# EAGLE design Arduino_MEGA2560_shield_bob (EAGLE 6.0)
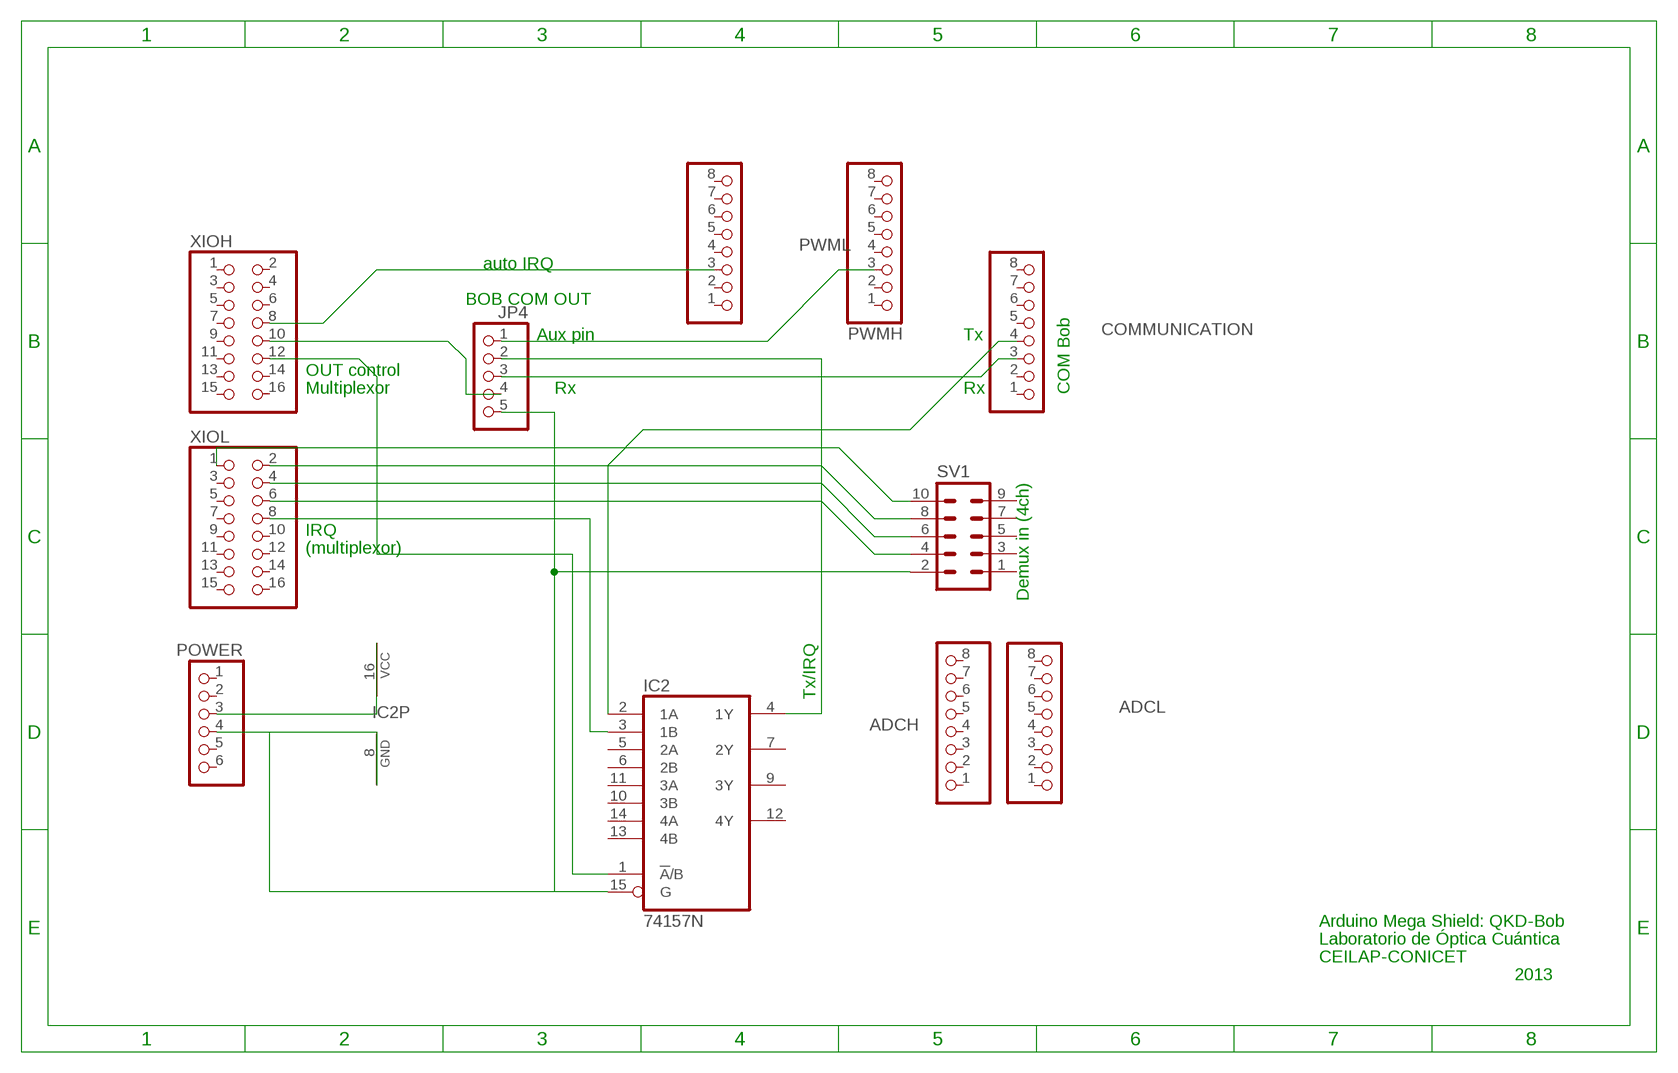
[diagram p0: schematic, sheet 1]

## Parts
ADCH  PINHD-1X8  [1X08]
ADCL  PINHD-1X8  [1X08]
COMMUNICATION  PINHD-1X8  [1X08]
IC2  74157N  [DIL16]
JP4  PINHD-1X5  [1X05]
POWER  PINHD-1X6  [1X06]
PWMH  PINHD-1X8  [1X08]
PWML  PINHD-1X8  [1X08]
SV1  ML10  [ML10]
XIOH  PINHD-2X8  [2X08]
XIOL  PINHD-2X8  [2X08]

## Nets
GND: IC2.8(GND) IC2.15(G) JP4.5 POWER.4 SV1.2
N$1: IC2.3(1B) XIOL.8
N$2: IC2.4(1Y) JP4.2
N$3: IC2.1(!A!/B) XIOH.12
N$4: IC2.16(VCC) POWER.3
N$5: SV1.10 XIOL.1
N$6: JP4.4 XIOH.10
N$7: JP4.1 PWMH.3
N$8: SV1.8 XIOL.2
N$9: COMMUNICATION.4 IC2.2(1A)
N$10: COMMUNICATION.3 JP4.3
N$11: SV1.6 XIOL.4
N$12: SV1.4 XIOL.6
N$13: PWML.3 XIOH.8
Unconnected: ADCH.1 ADCH.2 ADCH.3 ADCH.4 ADCH.5 ADCH.6 ADCH.7 ADCH.8 ADCL.1 ADCL.2 ADCL.3 ADCL.4 ADCL.5 ADCL.6 ADCL.7 ADCL.8 COMMUNICATION.1 COMMUNICATION.2 COMMUNICATION.5 COMMUNICATION.6 COMMUNICATION.7 COMMUNICATION.8 IC2.5(2A) IC2.6(2B) IC2.7(2Y) IC2.9(3Y) IC2.10(3B) IC2.11(3A) IC2.12(4Y) IC2.13(4B) IC2.14(4A) POWER.1 POWER.2 POWER.5 POWER.6 PWMH.1 PWMH.2 PWMH.4 PWMH.5 PWMH.6 PWMH.7 PWMH.8 PWML.1 PWML.2 PWML.4 PWML.5 PWML.6 PWML.7 PWML.8 SV1.1 SV1.3 SV1.5 SV1.7 SV1.9 XIOH.1 XIOH.2 XIOH.3 XIOH.4 XIOH.5 XIOH.6 XIOH.7 XIOH.9 XIOH.11 XIOH.13 XIOH.14 XIOH.15 XIOH.16 XIOL.3 XIOL.5 XIOL.7 XIOL.9 XIOL.10 XIOL.11 XIOL.12 XIOL.13 XIOL.14 XIOL.15 XIOL.16

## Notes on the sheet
- auto IRQ
- BOB COM OUT
- Aux pin | Tx
- OUT control
- Multiplexor | Rx | Rx | COM Bob
- Demux in (4ch)
- IRQ
- (multiplexor)
- Tx/IRQ
- Arduino Mega Shield: QKD-Bob
- Laboratorio de Óptica Cuántica
- CEILAP-CONICET
- 2013

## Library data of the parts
ADCH ADCL COMMUNICATION PWMH PWML = pinhead:PINHD-1X8: PIN HEADER
IC2 = 74xx-us:74*157: Quadruple 2-line to 1-line data SELECTOR/MULTIPLEXER
JP4 = pinhead:PINHD-1X5: PIN HEADER
POWER = pinhead:PINHD-1X6: PIN HEADER
SV1 = con-harting-ml:ML10: HARTING; OC_FARNELL: unknown; OC_NEWARK: unknown
XIOH XIOL = pinhead:PINHD-2X8: PIN HEADER

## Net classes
0 default: width 0.152 mm, drill 0.305 mm, clearance 0.152 mm

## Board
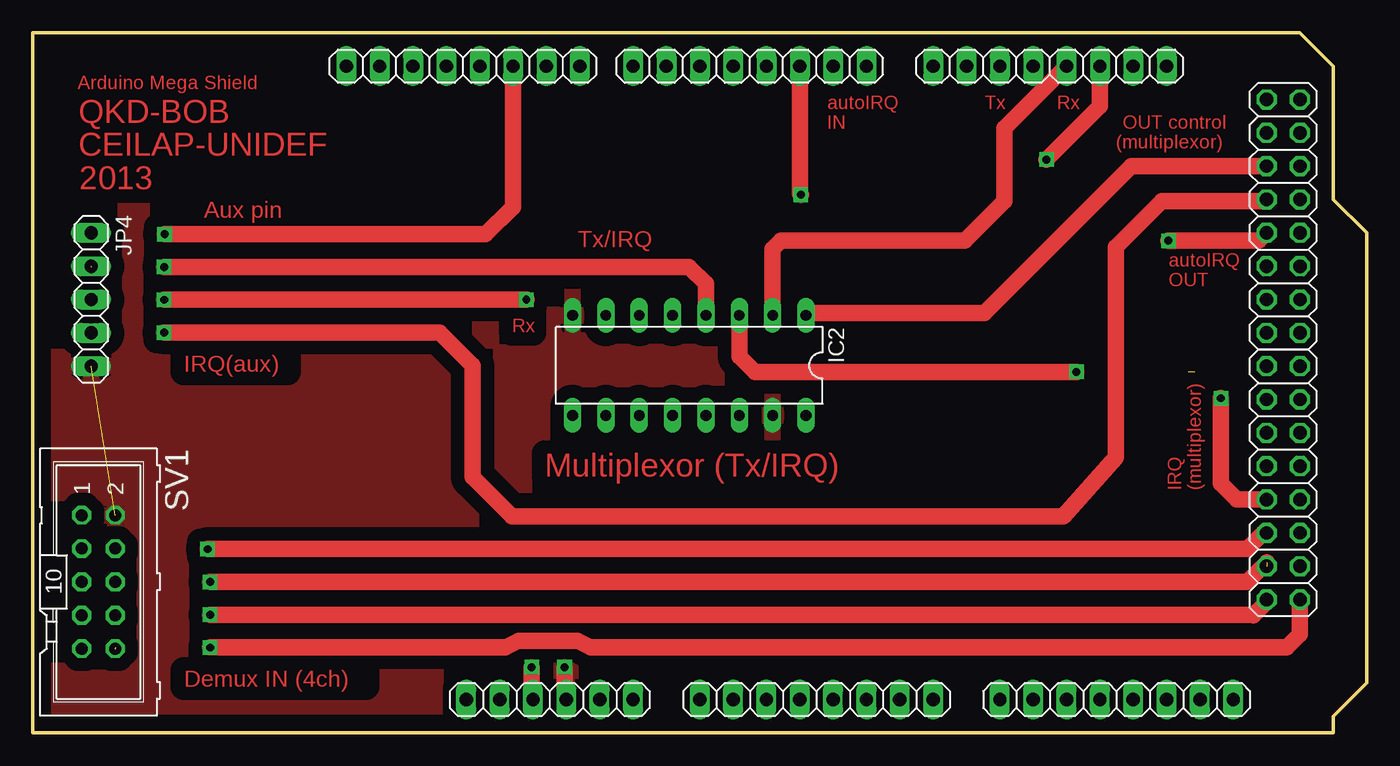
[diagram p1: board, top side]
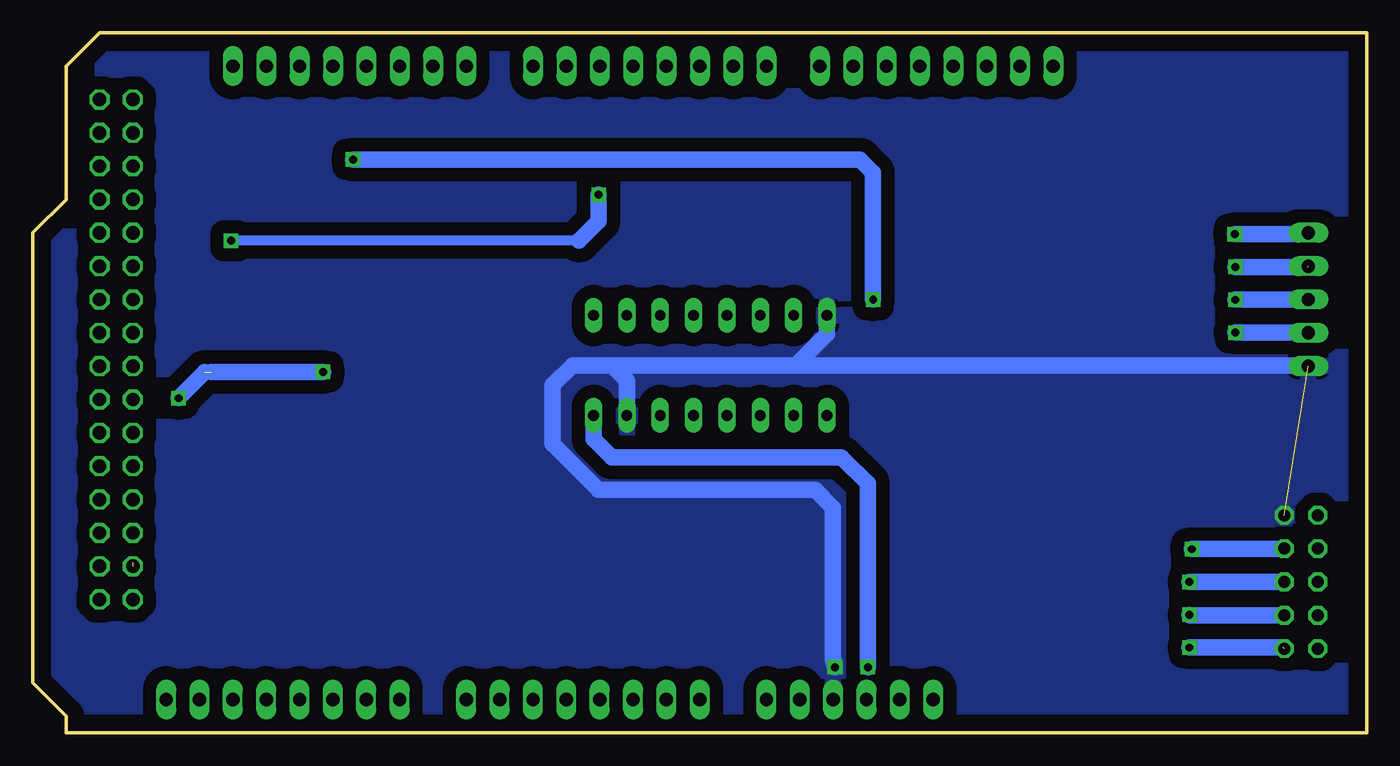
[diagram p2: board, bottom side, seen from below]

Size 101.6 x 53.34 mm. Coordinates in mm from the lower left corner, seen from the top.
Outline: 0,53.34 96.52,53.34 99.06,50.8 99.06,40.64 101.6,38.1 101.6,3.81 99.06,1.27 99.06,0 0,0 0,53.34
Copper layers (1*16): Top 0.035mm / dielectric 1.5mm / Bottom 0.035mm
Design rules: minimum track width 6mil, minimum drill 12mil, track to track 40mil, track to pad 20mil, pad to pad 10mil, via to via 6mil, smd to smd 6mil, copper to edge 50mil, drill to drill 12mil, minimum pad ring 10mil, minimum via ring 10mil, stop-mask expansion 5mil, vias tented up to drill 1mil, thermal gap 10mil

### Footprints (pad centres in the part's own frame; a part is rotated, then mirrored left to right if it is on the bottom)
1X08 = drill 1.016 long: 1 -8.89,0; 2 -6.35,0; 3 -3.81,0; 4 -1.27,0; 5 1.27,0; 6 3.81,0; 7 6.35,0; 8 8.89,0
DIL16 = drill 0.813 long: 1 -8.89,-3.81; 2 -6.35,-3.81; 3 -3.81,-3.81; 4 -1.27,-3.81; 5 1.27,-3.81; 6 3.81,-3.81; 7 6.35,-3.81; 8 8.89,-3.81; 9 8.89,3.81; 10 6.35,3.81; 11 3.81,3.81; 12 1.27,3.81; 13 -1.27,3.81; 14 -3.81,3.81; 15 -6.35,3.81; 16 -8.89,3.81
1X05 = drill 1.016 long: 1 -5.08,0; 2 -2.54,0; 3 0,0; 4 2.54,0; 5 5.08,0
1X06 = drill 1.016 long: 1 -6.35,0; 2 -3.81,0; 3 -1.27,0; 4 1.27,0; 5 3.81,0; 6 6.35,0
ML10 = drill 0.914 octagon: 1 -5.08,-1.27; 2 -5.08,1.27; 3 -2.54,-1.27; 4 -2.54,1.27; 5 0,-1.27; 6 0,1.27; 7 2.54,-1.27; 8 2.54,1.27; 9 5.08,-1.27; 10 5.08,1.27
2X08 = drill 1.016 octagon: 1 -8.89,-1.27; 2 -8.89,1.27; 3 -6.35,-1.27; 4 -6.35,1.27; 5 -3.81,-1.27; 6 -3.81,1.27; 7 -1.27,-1.27; 8 -1.27,1.27; 9 1.27,-1.27; 10 1.27,1.27; 11 3.81,-1.27; 12 3.81,1.27; 13 6.35,-1.27; 14 6.35,1.27; 15 8.89,-1.27; 16 8.89,1.27

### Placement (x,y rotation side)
ADCH  82.55,2.54 0 top
ADCL  59.69,2.54 0 top
COMMUNICATION  77.47,50.8 180 top
IC2  50,28 180 top
JP4  4.45,33.02 270 top
POWER  39.37,2.54 0 top
PWMH  32.77,50.8 180 top
PWML  54.61,50.8 180 top
SV1  5,11.5 270 top
XIOH  95.25,39.37 90 top
XIOL  95.25,19.05 90 top

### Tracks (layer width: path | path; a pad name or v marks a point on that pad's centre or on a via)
GND  (via drill 0.6)  (1 unrouted)
  Top 1.27: v40.5,5 40.5,3.18 POWER.4
  Bottom 1.27: 57.5,28 60.5,28 62,26.5 62,22 58.5,18.5 42,18.5 40.64,17.14 40.64,5.64 v40.5,5 | 43.5,28 57.5,28 | IC2.15 56.35,26.85 57.5,28 | IC2.8 41.11,30.39 43.5,28 | 43.5,28 4.5,28 JP4.5
  pour Top: 0.02,52.83 96.52,52.83 98.55,50.8 98.55,41.66 101.6,38.61 101.6,4.06 98.55,1.02 98.55,0 0,0
  pour Bottom: 0.02,52.83 96.52,52.83 98.55,50.8 98.55,41.66 101.6,38.61 101.6,4.06 98.55,1.02 98.55,0 0,0
N$1  (via drill 0.6)  (1 unrouted)
  Top 1.27: IC2.3 53.81,28.69 55,27.5 v79.5,27.5 | XIOL.8 91.72,17.78 90.5,19 v90.5,25.5
  Bottom 1.27: v79.5,27.5 88,27.5 | v90.5,25.5 | v90.5,25.5 88.5,27.5
N$2  (via drill 0.6)  (1 unrouted)
  Top 1.27: IC2.4 51.27,34.23 50,35.5 v10,35.5
  Bottom 1.27: 4.5,35.5 v10,35.5 | v10,35.5
N$3
  Top 1.27: IC2.1 59.08,32 72.5,32 83.68,43.18 XIOH.12
N$4  (via drill 0.6)
  Top 1.27: v38,5 38,2.64 POWER.3
  Bottom 1.27: 38,5.5 38,19 40,21 57.5,21 58.89,22.39 IC2.16 | 38,5.14 38,5.5 | 38,5.5 v38,5
N$5  (via drill 0.6)  (1 unrouted)
  Top 1.27: v13.5,6.5 35.5,6.5 36,6.5 37,7 41.5,7 42.5,6.5 95.5,6.5 96.5,7.5 96.5,10.14 XIOL.1
  Bottom 1.27: 6.35,6.5 v13.5,6.5 | v13.5,6.5
N$6  (via drill 0.6)  (1 unrouted)
  Top 1.27: JP4.4 4.46,30.5 | XIOH.10 93.84,40.5 86,40.5 82.5,37 82.5,36 82.5,21 78.5,16.5 62,16.5 36.5,16.5 33.5,19.5 | 33.5,19.5 33.5,28 31,30.5 v10,30.5 | 33.5,19.5
  Bottom 1.27: v10,30.5 4.46,30.5 JP4.4
N$7  (via drill 0.6)
  Top 1.27: v10.04,38 34.5,38 36.58,40.08 PWMH.3
  Bottom 1.27: v10.04,38 4.54,38 JP4.1
N$8  (via drill 0.6)
  Top 1.27: 92.96,8.96 93,9 | XIOL.2 93.98,9.98 93.25,9.25 93,9 | v13.5,9 93,9
  Bottom 1.27: SV1.8 13.46,8.96 v13.5,9
N$9
  Top 1.27: COMMUNICATION.4 74,46.06 74,40.5 71,37.5 57,37.5 56.35,36.85 IC2.2
N$10  (via drill 0.6)
  Top 1.27: v77.22,43.69 81.28,47.75 COMMUNICATION.3 | v10,33 37.1,33 v37.59,33.01
  Bottom 1.27: v37.59,33.01 37.59,42.67 38.61,43.69 v77.22,43.69 | JP4.3 9.98,33.02 v10,33
N$11  (via drill 0.6)  (1 unrouted)
  Top 1.27: 92.5,11.5 94,13 | v13.5,11.5 92.5,11.5 | 92.5,11.5
  Bottom 1.27: SV1.6 v13.5,11.5 | v13.5,11.5
N$12  (via drill 0.6)
  Top 1.27: v13.31,14 92.5,14 93.74,15.24 XIOL.6
  Bottom 1.27: v13.31,14 6.31,14 SV1.4
N$13  (via drill 0.6)
  Top 1.27: PWML.3 58.42,41.08 v58.5,41 | v86.5,37.5 93.38,37.5 XIOH.8
  Bottom 0.762: 60,37.5 v86.5,37.5
  Bottom 1.27: v58.5,41 58.5,39 60,37.5

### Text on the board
Top: Arduino Mega Shield | autoIRQ | Tx | Rx | QKD-BOB | IN | OUT control | CEILAP-UNIDEF | (multiplexor) | 2013 | Aux pin | Tx/IRQ | autoIRQ | OUT | Rx | IRQ(aux) | Multiplexor (Tx/IRQ) | IRQ | (multiplexor) | Demux IN (4ch)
